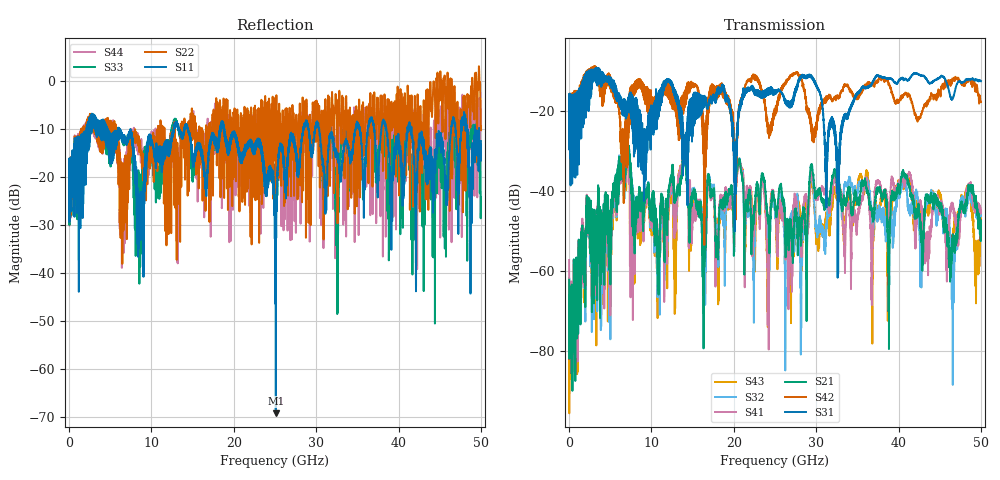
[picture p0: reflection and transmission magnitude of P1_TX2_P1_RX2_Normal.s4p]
!Keysight Technologies,N5225B,MY57041031,A.13.20.10
!Date: Friday, May 31, 2019 11:15:30
!Correction: S11(Full 4 Port(1,2,3,4))
!S12(Full 4 Port(1,2,3,4))
!S13(Full 4 Port(1,2,3,4))
!S14(Full 4 Port(1,2,3,4))
!S21(Full 4 Port(1,2,3,4))
!S22(Full 4 Port(1,2,3,4))
!S23(Full 4 Port(1,2,3,4))
!S24(Full 4 Port(1,2,3,4))
!S31(Full 4 Port(1,2,3,4))
!S32(Full 4 Port(1,2,3,4))
!S33(Full 4 Port(1,2,3,4))
!S34(Full 4 Port(1,2,3,4))
!S41(Full 4 Port(1,2,3,4))
!S42(Full 4 Port(1,2,3,4))
!S43(Full 4 Port(1,2,3,4))
!S44(Full 4 Port(1,2,3,4))
!S4P File: Measurements: <S11,S12,S13,S14>,
!<S21,S22,S23,S24>,
!<S31,S32,S33,S34>,
!<S41,S42,S43,S44>:
# Hz S  dB  R 50.0
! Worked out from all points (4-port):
!   5000 points, 10 MHz to 50 GHz, reference 50 ohm
!   strongest paths, dB at 10 MHz, 12.51 GHz, 25.01 GHz, 37.51 GHz, 50 GHz:
!     S31: -19.5, -13.0, -15.4, -11.1, -12.5
!     S42: -19.3, -16.4, -19.4, -12.5, -17.7
!     S21: -62.2, -34.9, -43.3, -39.8, -51.0
!     S41: -57.2, -37.7, -43.4, -37.5, -45.6
!     S32: -69.1, -37.4, -45.2, -45.3, -45.7
!     S43: -61.9, -40.2, -44.7, -45.9, -46.5
!   lowest |S11| = -69.2 dB at 25.1 GHz (marker M1), VSWR 1.00, Z = 50 - j0.0107 ohm
!   |S11| at or under -10 dB: 6.091 GHz to 12.71 GHz (6.616 GHz wide, 70.4 % of centre); 18.82 GHz to 28.43 GHz (9.605 GHz wide, 40.7 % of centre); 41.58 GHz to 46.39 GHz (4.81 GHz wide, 10.9 % of centre)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
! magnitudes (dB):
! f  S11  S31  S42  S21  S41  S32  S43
! 10 MHz  -19.8  -19.5  -19.3  -62.2  -57.2  -69.1  -61.9
! 7.15 GHz  -12.2  -19.4  -33.2  -29.7  -31.8  -29.4  -31.1
! 10.84 GHz  -14.7  -16.5  -17.6  -59.6  -56.0  -56.9  -62.7
! 13.98 GHz  -10.7  -30.9  -16.7  -30.3  -29.2  -30.6  -29.9
! 25.1 GHz  -69.2  -15.1  -19.2  -44.3  -45.0  -46.1  -46.6
! 32.64 GHz  -15.8  -37.2  -16.3  -37.6  -39.9  -37.9  -41.5
! 50 GHz  -12.6  -12.5  -17.7  -51.0  -45.6  -45.7  -46.5
